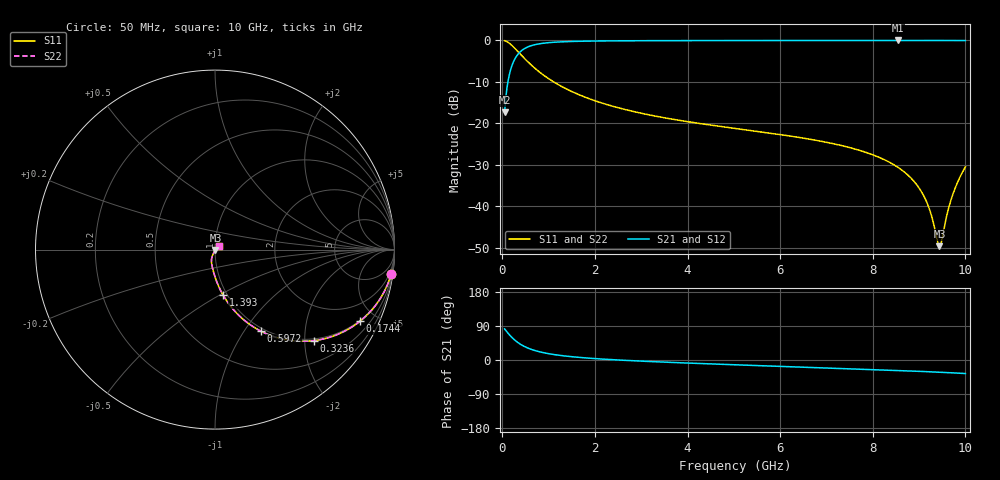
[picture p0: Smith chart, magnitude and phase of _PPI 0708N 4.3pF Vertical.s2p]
! S-Parameter data specifications (vertical orientation):
! Substrate: 40-mil Rogers 3003C, Substrate thickness, H=1.016mm, Dielectric constant, Er=3, Conductor thickness, T_mtl=0.043mm, Loss Tangent, Tand=0.003
! PCB Mounting Pad Footprint: Pad width, PadW=2.54mm , Pad length, PadL=0.51mm , Pad gap, PadG (edge-to-edge)=0.71mm , Reference planes=1.73mm apart
! Created Tue Jan 16 08:45:28 2018
# GHz S MA R 50
! 2 Port Network Data from SP1.SP block
! freq  magS11  angS11  magS21  angS21  magS12  angS12  magS22  angS22
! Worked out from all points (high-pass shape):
!   801 points, 50 MHz to 10 GHz, reference 50 ohm
!   highest |S21| = -0.03 dB at 8.545 GHz (marker M1); lowest = -17.3 dB at 50 MHz (marker M2)
!   |S21| within 3 dB of the highest: 363.3 MHz to end of sweep
!   lowest |S11| = -49.6 dB at 9.44 GHz (marker M3), VSWR 1.01, Z = 50.3 - j0.196 ohm
!   |S11| at or under -10 dB: 1.108 GHz to end of sweep
!   |S22| runs from -49.6 to -0.1 dB; largest |S21 - S12| = 0
!   S11 on the Smith chart (normalised r, x): 50 MHz: 1, -14; 174.4 MHz: 0.96, -4.08; 323.6 MHz: 0.96, -2.20; 597.2 MHz: 0.96, -1.20; 1.393 GHz: 0.96, -0.52; 10 GHz: 1.04, +0.04
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0.05  0.9907 -8.0  0.1361 82.0  0.1361 82.0  0.9907 -8.0
0.174375  0.9018 -26.2  0.432 63.8  0.432 63.8  0.9018 -26.2
0.323625  0.7475 -42.8  0.6639 47.2  0.6639 47.2  0.7475 -42.8
0.59725  0.5218 -60.6  0.8526 29.3  0.8526 29.3  0.5218 -60.6
0.9081875  0.3751 -71.1  0.9264 18.8  0.9264 18.8  0.3751 -71.1
1.39325  0.2583 -79.8  0.9654 10.0  0.9654 10.0  0.2583 -79.8
1.716625  0.2145 -83.5  0.9759 6.3  0.9759 6.3  0.2145 -83.5
3.370812  0.1203 -94.5  0.9916 -5.0  0.9916 -5.0  0.1203 -94.5
5.025  0.08697 -101.8  0.9948 -12.6  0.9948 -12.6  0.08697 -101.8
6.691625  0.0637 -108.2  0.9961 -19.6  0.9961 -19.6  0.0637 -108.2
7.66175  0.04826 -111.5  0.9967 -23.7  0.9967 -23.7  0.04826 -111.5
8.345812  0.03433 -113.1  0.9969 -26.8  0.9969 -26.8  0.03433 -113.1
8.544813  0.02951 -113.2  0.9969 -27.7  0.9969 -27.7  0.02951 -113.2
8.85575  0.02105 -112.2  0.9969 -29.2  0.9969 -29.2  0.02105 -112.2
9.079625  0.0141 -108.9  0.9967 -30.3  0.9967 -30.3  0.0141 -108.9
9.228875  0.009072 -101.9  0.9966 -31.1  0.9966 -31.1  0.009072 -101.9
9.390562  0.003955 -67.3  0.9964 -32.0  0.9964 -32.0  0.003955 -67.3
9.440312  0.003317 -36.0  0.9963 -32.2  0.9963 -32.2  0.003317 -36.0
9.490063  0.00391 -3.0  0.9962 -32.5  0.9962 -32.5  0.00391 -3.0
9.614437  0.008475 31.2  0.9959 -33.2  0.9959 -33.2  0.008475 31.2
9.726375  0.01385 39.6  0.9956 -33.9  0.9956 -33.9  0.01385 39.6
10  0.02991 45.0  0.9944 -35.7  0.9944 -35.7  0.02991 45.0
